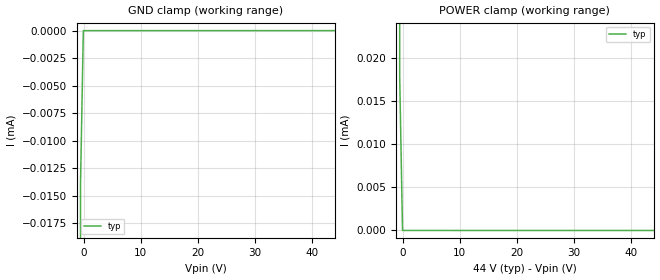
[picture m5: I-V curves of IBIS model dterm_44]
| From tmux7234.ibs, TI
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| dterm_44
[Model]   dterm_44
Model_type   Terminator
|   typ   min   max
C_comp   1.598234e-11   NA   NA
[Voltage Range]   44   NA   NA
[Temperature Range]   27   NA   NA
[Power Clamp Reference]   44   NA   NA
[GND Clamp Reference]   0   NA   NA
[GND Clamp]
|   Voltage   I(typ)   I(min)   I(max)
-5V       -2.391A    NA         NA
-1.04V    -70.51mA   NA         NA
-545.5mV  -13.98uA   NA         NA
-50.51mV  -1.467nA   NA         NA
44V       1.409nA    NA         NA
[POWER Clamp]
|   Voltage   I(typ)   I(min)   I(max)
-5V       3.083A     NA         NA
-1.04V    72.32mA    NA         NA
-545.5mV  17.87uA    NA         NA
-50.5mV   1.416nA    NA         NA
44V       -1.456nA   NA         NA
